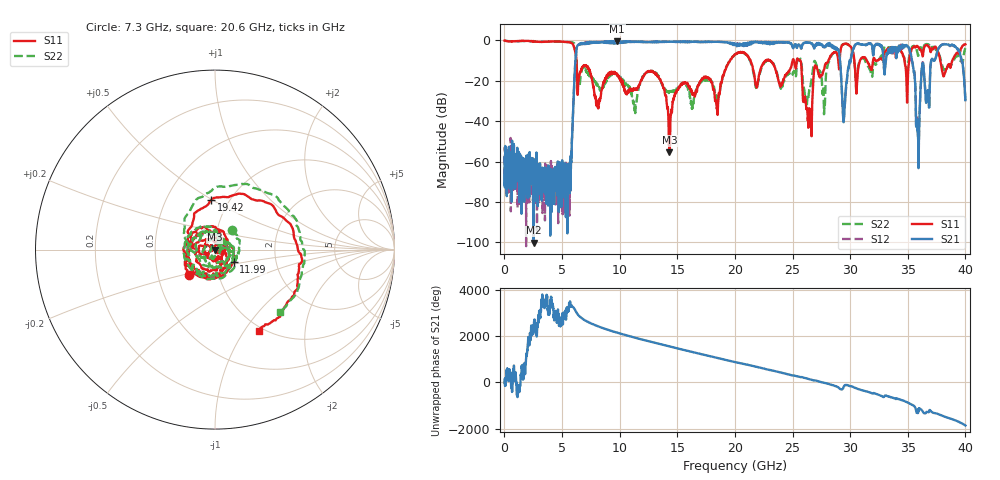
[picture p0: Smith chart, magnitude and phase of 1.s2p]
! 4/12/2023 4:22:52 PM
! D:\_XLC\ZHPF1-M6.3-18G-450\1.S2P
! CHANNEL.1
! TR.MEASUREMENT
! CORRECTED.DATA
! RF.CORRECTION: FULL.TWO.PORT.CAL.PORT.1.2
! AVERAGING.OFF
! IF.BANDWIDTH: 100KHZ
! SWEEPTYPE:  FREQ.SWEEP(Linear)
! Reference Plane Port Info
! PORT:  PORT1  PORT2
! DISTANCE:  0  m  0  m
! TIME:  0  s  0  s
! PHASE.OFFSET:  0 °  0 °
! LOSS:  0  dB  0  dB
! REF.LOSS:  0  dB  0  dB
! REF.FREQ:  0  Hz  0  Hz
! Power Info
! POWER:  -10  dBm  -10  dBm
! EFF.POWER:  -10  dBm  -10  dBm
! SOURCE.ATTEN:  0  dB  0  dB
! TEST.ATTEN:  0  dB  0  dB
# GHZ S RI R 50.0
! FREQ.GHZ  S11RE  S11IM  S21RE  S21IM  S12RE  S12IM  S22RE  S22IM
!; PortSelection: Port_12
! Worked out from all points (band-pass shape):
!   4000 points, 10 MHz to 40 GHz, reference 50 ohm
!   highest |S21| = -0.39 dB at 9.79 GHz (marker M1); lowest = -100.1 dB at 2.52 GHz (marker M2)
!   |S21| within 3 dB of the highest: 6.275 GHz to 25.02 GHz (18.74 GHz wide, 120 % of centre); 30.34 GHz to 31.93 GHz (1.589 GHz wide, 5.1 % of centre)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
!   lowest |S11| = -55.4 dB at 14.31 GHz (marker M3), VSWR 1.00, Z = 49.8 - j0.051 ohm
!   |S11| at or under -10 dB: 6.247 GHz to 19.56 GHz (13.32 GHz wide, 103 % of centre); 23.08 GHz to 25 GHz (1.92 GHz wide, 7.99 % of centre); 25.63 GHz to 28.11 GHz (2.479 GHz wide, 9.23 % of centre)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
!   |S22| runs from -36.5 to 0.0 dB; largest |S21 - S12| = 0.16
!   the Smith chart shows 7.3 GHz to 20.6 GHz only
!   S11 on the Smith chart (normalised r, x): 7.3 GHz: 0.72, -0.21; 11.99 GHz: 1.22, -0.17; 19.42 GHz: 0.82, +0.49; 20.6 GHz: 0.95, -1.17
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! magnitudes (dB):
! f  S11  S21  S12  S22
! 10 MHz  0.0  -72.2  -67.7  0.0
! 2.52 GHz  -0.6  -100.1  -67.3  -0.5
! 5.55 GHz  -0.8  -61.2  -85.7  -0.8
! 6.22 GHz  -7.9  -5.4  -5.5  -6.9
! 6.68 GHz  -14.1  -1.5  -1.3  -15.5
! 7.3 GHz  -13.9  -1.1  -1.0  -16.7
! 9.79 GHz  -16.9  -0.4  -0.9  -17.2
! 11.99 GHz  -18.0  -0.8  -0.6  -17.7
! 13.34 GHz  -17.9  -0.8  -0.9  -17.6
! 14.31 GHz  -55.4  -0.6  -0.7  -25.3
! 19.42 GHz  -11.2  -1.0  -1.1  -11.4
! 20.01 GHz  -7.0  -2.3  -2.1  -7.0
! 20.6 GHz  -5.7  -2.0  -2.3  -6.0
! 26.67 GHz  -39.8  -1.3  -1.6  -18.5
! 28.89 GHz  -7.2  -4.2  -3.9  -6.1
! 29.45 GHz  -1.8  -39.0  -39.1  -1.7
! 30.46 GHz  -17.0  -2.0  -2.0  -18.1
! 33.34 GHz  -3.8  -5.1  -4.9  -3.6
! 35.12 GHz  -10.3  -4.1  -4.3  -8.2
! 35.87 GHz  -3.0  -45.2  -45.5  -7.2
! 37.94 GHz  -13.8  -2.2  -2.2  -11.3
! 40 GHz  -1.9  -29.6  -29.9  -3.8
